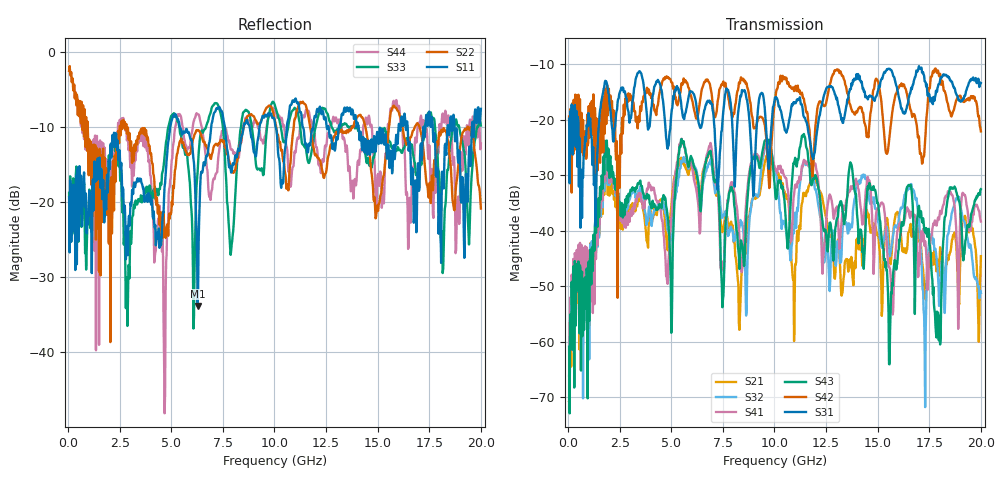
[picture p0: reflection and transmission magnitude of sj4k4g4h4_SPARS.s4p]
! FILE: E:\users\goganessyan\GBX_Backplane\FR408_backplane\1m_INBOUND_NEXT\sj4k4g4h4_SPARS.s4p
# MHZ S RI R 50.00
! FREQ  S11  S12  S13  S14
!  S21  S22  S23  S24
!  S31  S32  S33  S34
!  S41  S42  S43  S44
!  REAL  IMAG  REAL  IMAG  REAL  IMAG  REAL  IMAG
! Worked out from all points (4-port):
!   799 points, 50 MHz to 20 GHz, reference 50 ohm
!   strongest paths, dB at 50 MHz, 5.025 GHz, 10.03 GHz, 15.03 GHz, 20 GHz:
!     S31: -19.8, -18.1, -16.0, -14.7, -13.4
!     S42: -19.4, -13.3, -16.4, -13.2, -22.1
!     S43: -60.9, -56.9, -32.5, -35.2, -32.5
!     S41: -71.9, -37.2, -28.7, -35.8, -38.3
!     S32: -66.1, -39.3, -28.8, -38.4, -51.2
!     S21: -70.8, -34.4, -28.9, -40.6, -44.6
!   lowest |S11| = -33.8 dB at 6.275 GHz (marker M1), VSWR 1.04, Z = 51.6 - j1.33 ohm
!   |S11| at or under -10 dB: start of sweep to 4.947 GHz; 5.415 GHz to 6.932 GHz (1.517 GHz wide, 24.6 % of centre); 14.08 GHz to 16.01 GHz (1.933 GHz wide, 12.8 % of centre)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
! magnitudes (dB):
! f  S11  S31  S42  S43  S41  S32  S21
! 50 MHz  -19.3  -19.8  -19.4  -60.9  -71.9  -66.1  -70.8
! 1.875 GHz  -16.6  -13.4  -14.2  -23.7  -24.9  -26.0  -27.2
! 4.675 GHz  -18.0  -19.4  -12.7  -34.3  -43.1  -35.6  -37.3
! 6.275 GHz  -33.8  -18.9  -19.4  -30.6  -34.2  -30.2  -31.9
! 16.55 GHz  -12.0  -15.3  -17.6  -31.7  -37.4  -32.0  -39.6
! 17.98 GHz  -22.3  -13.5  -12.1  -59.8  -37.9  -53.5  -48.1
! 20 GHz  -7.6  -13.4  -22.1  -32.5  -38.3  -51.2  -44.6
